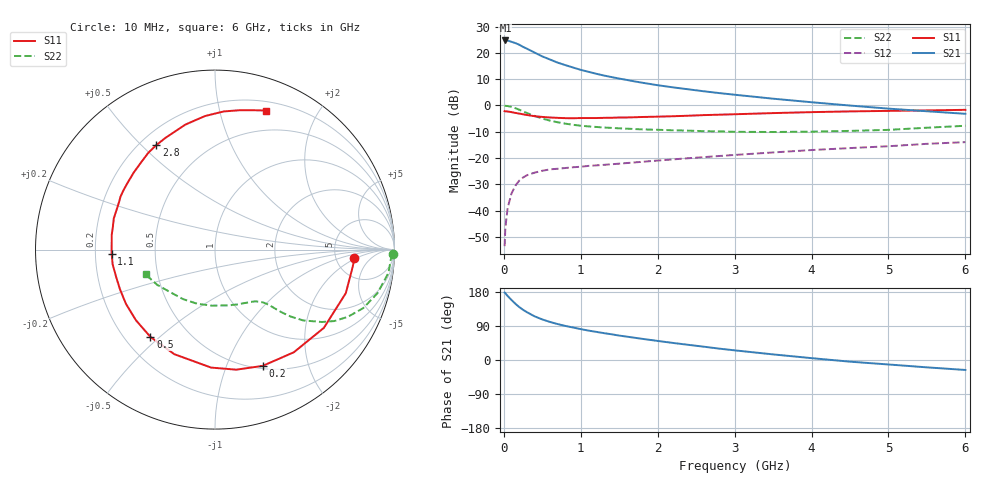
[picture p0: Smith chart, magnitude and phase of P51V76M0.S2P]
! SIEMENS Small Signal Semiconductors
! BFP183
! Si NPN RF Bipolar Junction Transistor in SOT143
! VCE = 1.75 V  IC = 6 mA
! Common Emitter S-Parameters:  March  1996
# GHz  S  MA  R  50
!  f  S11  S21  S12  S22
! GHz  MAG  ANG  MAG  ANG  MAG  ANG  MAG  ANG
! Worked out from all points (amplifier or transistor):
!   36 points, 10 MHz to 6 GHz, reference 50 ohm
!   highest |S21| = 24.7 dB at 20 MHz (marker M1)
!   |S21| within 3 dB of that: start of sweep to 290.3 MHz
!   unconditionally stable (mu >= 1): 1.411 GHz to 5.744 GHz
!   at 250 MHz: K = 0.24, MSG = 24.9 dB, |S12| = -27.4 dB
!   at 1.4 GHz: K = 1.00, MSG = 16.6 dB, |S12| = -22.4 dB
!   at 6 GHz: K = 0.96, MSG = 5.4 dB, |S12| = -14.0 dB
!   S11 on the Smith chart (normalised r, x): 10 MHz: 7.56, -1.88; 200 MHz: 0.53, -1.35; 500 MHz: 0.30, -0.47; 1.1 GHz: 0.27, -0.02; 2.8 GHz: 0.26, +0.55; 6 GHz: 0.29, +1.40
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0.01  0.7786 -3.6  17.21 178.0  0.0021 87.3  0.992 -1.5
0.02  0.7725 -7.5  17.27 175.9  0.0048 87.6  0.9814 -3.1
0.05  0.7682 -18.4  17.18 168.8  0.0113 82.5  0.975 -7.7
0.1  0.7471 -35.7  16.26 158.3  0.0212 71.9  0.9368 -15.1
0.15  0.7212 -52.5  15.39 148.4  0.0298 64.5  0.8883 -21.5
0.2  0.7002 -67.7  14.33 139.7  0.0371 58.4  0.8301 -26.8
0.25  0.6793 -80.0  13.03 132.4  0.0426 53.0  0.775 -30.9
0.3  0.6577 -91.9  12.04 126.2  0.047 49.1  0.7195 -34.1
0.4  0.6252 -111.3  10.15 115.2  0.0527 42.9  0.6296 -38.8
0.5  0.605 -126.5  8.58 107.0  0.0572 38.5  0.5628 -41.5
0.6  0.5908 -138.2  7.49 100.4  0.0608 35.9  0.5146 -43.1
0.7  0.581 -148.7  6.534 94.8  0.0625 34.6  0.4784 -44.2
0.9  0.5715 -164.5  5.273 85.7  0.0667 33.2  0.4286 -45.9
1.1  0.5764 -177.8  4.372 77.6  0.0708 32.6  0.3994 -47.6
1.5  0.59 162.8  3.25 64.4  0.0781 33.1  0.3671 -51.8
1.8  0.6036 150.7  2.71 55.8  0.0847 34.0  0.3505 -56.1
2.2  0.6239 136.6  2.21 45.0  0.0942 34.2  0.3365 -63.0
2.8  0.6675 119.3  1.721 30.0  0.1092 33.3  0.3212 -75.7
3.5  0.7159 103.3  1.346 14.8  0.1276 31.3  0.3127 -93.3
4.5  0.7712 86.4  0.996 -4.4  0.1545 26.1  0.3282 -122.7
5.5  0.8055 74.6  0.776 -19.4  0.1862 20.3  0.3772 -148.6
6  0.8259 69.7  0.694 -26.3  0.2006 16.3  0.4109 -160.3
